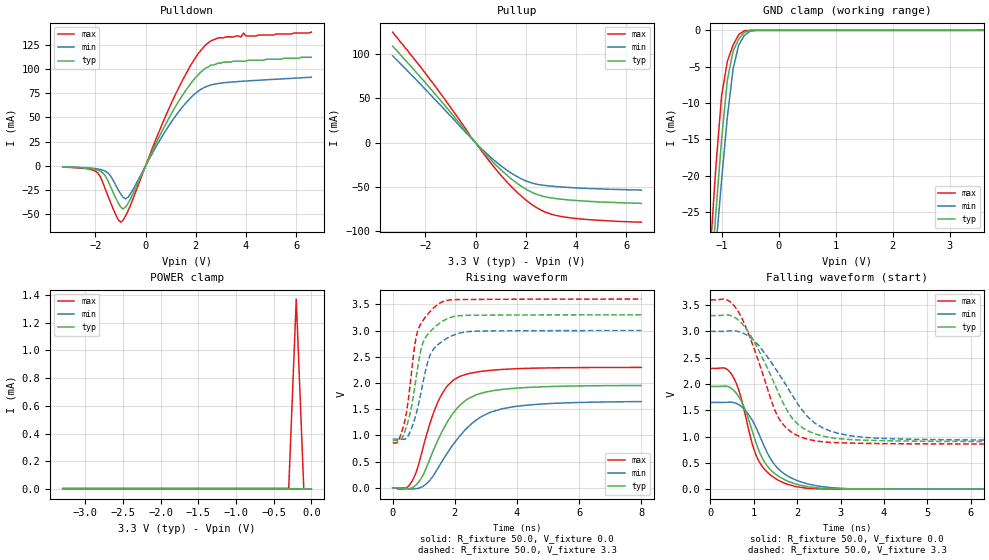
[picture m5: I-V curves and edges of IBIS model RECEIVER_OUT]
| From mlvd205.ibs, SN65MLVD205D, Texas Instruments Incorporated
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|   Receiver Output Model
[Model]   RECEIVER_OUT
Model_type   3-state
| Signals   R
Vmeas = 1.5V   |Reference voltage for timing measurements
Cref = 5pF   |Timing specification test load capacitance value
Vref = 0   |Timing specification test load voltage; GND
| variable   typ   min   max
C_comp   6.76pF   6.06pF   7.50pF
|   typ   min   max
[Temperature Range]   25.0   85   -40
[Voltage range]   3.3V   3.0V   3.6V
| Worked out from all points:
|   slope of the pulldown table from 0 to 0.495 V, typ, clamps not added: 18 ohm
|   slope of the pullup table from 0 to 0.495 V, typ, clamps not added: 31.2 ohm
|   GND clamp passes 1 mA (typ) near -0.68 V on its own axis
|   rising waveform, R_fixture 50.0, V_fixture 0.0: 20-80 % time 1.05ns typ, 1.34ns min, 795ps max; typ from 0 V to 1.95 V
|   falling waveform, R_fixture 50.0, V_fixture 0.0: 20-80 % time 587ps typ, 683ps min, 502ps max; typ from 1.95 V to 0 V
|   rising waveform, R_fixture 50.0, V_fixture 3.3: 20-80 % time 469ps typ, 528ps min, 409ps max; typ from 0.903 V to 3.3 V
|   falling waveform, R_fixture 50.0, V_fixture 3.3: 20-80 % time 860ps typ, 1.04ns min, 709ps max; typ from 3.3 V to 0.904 V
[Pulldown]
|   Voltage   I(typ)   I(min)   I(max)
-3.3V     -1.2mA     -1mA       -1.3mA
-1.9V     -4.4mA     -3.3mA     -7.4mA
-1.5V     -15.3mA    -7.29mA    -30.9mA
-1V       -42.1mA    -28.6mA    -58.1mA
-800mV    -42.7mA    -34mA      -51.7mA
-600mV    -34mA      -28.8mA    -40.5mA
400mV     22.3mA     19mA       26.7mA
1.2V      61.6mA     51.7mA     74.2mA
1.8V      85mA       70.3mA     104mA
2.4V      101mA      81.6mA     125mA
3.9V      108mA      87.4mA     137mA
6.6V      112mA      91.4mA     138mA
[Pullup]
|   Voltage   I(typ)   I(min)   I(max)
| Note that the[Pullup]voltage table is referenced to Vcc
| and is calculated using Vtable=Vcc - Vmeasured.
-3.3V     109mA      98.2mA     125mA
-1.7V     58mA       51.4mA     67.3mA
-300mV    10.2mA     8.89mA     12mA
-200mV    6.78mA     5.89mA     6.61mA
-100mV    3.37mA     2.92mA     3.98mA
400mV     -12.9mA    -11.1mA    -15.4mA
1.3V      -37.9mA    -32mA      -45.8mA
2.1V      -53.9mA    -44.1mA    -66.8mA
2.8V      -61.2mA    -48.3mA    -78.6mA
3.4V      -63.7mA    -49.9mA    -83.2mA
4.4V      -66mA      -51.5mA    -86.6mA
6.6V      -68.5mA    -53.5mA    -89.7mA
[GND_clamp]
|   Voltage   I(typ)   I(min)   I(max)
| Outputs in High Impedance (off)
-3.6V     -320mA     -293mA     -351mA
-1.2V     -35.7mA    -39.6mA    -30.4mA
-1.1V     -24.9mA    -29.8mA    -18.6mA
-1V       -14.9mA    -20.5mA    -8.91mA
-900mV    -6.84mA    -11.9mA    -4.26mA
-800mV    -2.89mA    -5.31mA    -2.04mA
-700mV    -1.18mA    -2.01mA    -577uA
-600mV    -262uA     -680uA     -52.8uA
-500mV    -21.7uA    -124uA     -1.49uA
-400mV    -918nA     -10.5uA    -18.3nA
3.6V      3.66uA     2.34uA     95.8nA
[POWER_clamp]
|   Voltage   I(typ)   I(min)   I(max)
| Note that the [POWER_clamp] voltage table is referenced to Vcc
| and is calculated using Vtable = Vcc - Vmeasured.
| Outputs in Tri-state.
-3.3V     3.67uA     2.35uA     6.42uA
-300mV    3.66uA     2.34uA     6.41uA
-200mV    3.66uA     2.35uA     1.37mA
-100mV    1.03uA     747nA      1.85uA
0V        60.9nA     55.9nA     95.8nA
[Ramp]
|   typ   min   max
dV/dt_r   1.171V/1.046ns   0.989V/1.342ns  1.378V/795ps
dV/dt_f   1.438V/860ps   1.243V/1.036ns  1.646V/709ps
R_load = 50
[Rising Waveform]
R_fixture = 50.0
V_fixture = 0.0
C_fixture = 0p
L_fixture = 0n
|   V(typ)   V(min)   V(max)
0s        0V         0V         0V
450ps     -23mV      -13mV      3mV
800ps     85mV       -12mV      377mV
1.2ns     555mV      146mV      1.23V
1.45ns    904mV      368mV      1.631V
1.75ns    1.249V     657mV      1.938V
2.15ns    1.569V     983mV      2.121V
2.8ns     1.794V     1.338V     2.217V
3.55ns    1.878V     1.511V     2.259V
8ns       1.951V     1.645V     2.296V
[Falling Waveform]
R_fixture = 50.0
V_fixture = 0.0
C_fixture = 0p
L_fixture = 0n
|   V(typ)   V(min)   V(max)
0s        1.952V     1.648V     2.297V
350ps     1.959V     1.65V      2.296V
500ps     1.91V      1.652V     2.172V
750ps     1.615V     1.546V     1.606V
950ps     1.151V     1.335V     909mV
1.1ns     774mV      1.089V     563mV
1.4ns     358mV      563mV      261mV
1.75ns    165mV      267mV      101mV
3.15ns    4mV        10mV       4mV
8ns       0V         0V         0V
[Rising Waveform]
R_fixture = 50.0
V_fixture = 3.3
V_fixture_min = 3.0
V_fixture_max = 3.6
C_fixture = 0p
L_fixture = 0n
|   V(typ)   V(min)   V(max)
0s        903mV      928mV      857mV
150ps     902mV      928mV      864mV
400ps     1.091V     928mV      1.304V
600ps     1.531V     1.129V     2.179V
800ps     2.28V      1.514V     2.985V
950ps     2.725V     1.935V     3.171V
1.15ns    2.943V     2.448V     3.326V
1.55ns    3.156V     2.776V     3.534V
2.55ns    3.291V     2.985V     3.592V
8ns       3.3V       3V         3.6V
[Falling Waveform]
R_fixture = 50.0
V_fixture = 3.3
V_fixture_min = 3.0
V_fixture_max = 3.6
C_fixture = 0p
L_fixture = 0n
|   V(typ)   V(min)   V(max)
0s        3.3V       3V         3.6V
450ps     3.305V     3.008V     3.569V
800ps     3.082V     2.948V     3.118V
1.1ns     2.663V     2.744V     2.46V
1.55ns    1.87V      2.23V      1.391V
1.8ns     1.453V     1.903V     1.129V
2.05ns    1.214V     1.578V     1.004V
2.6ns     1.009V     1.16V      901mV
3.25ns    941mV      1.013V     876mV
8ns       904mV      930mV      857mV
